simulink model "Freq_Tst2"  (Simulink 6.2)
settings: Solver=ode45  StartTime=0.0  StopTime=400  FixedStep=0.0005  MaxStep=0.002  RelTol=1e-3
undefined symbols (not defined in the file or in its folder): Aai, Aao, Af, Bai, Bao, Bf, Cai, Cao, Cf, Dai, Dao, Df, KJmix, KSmix

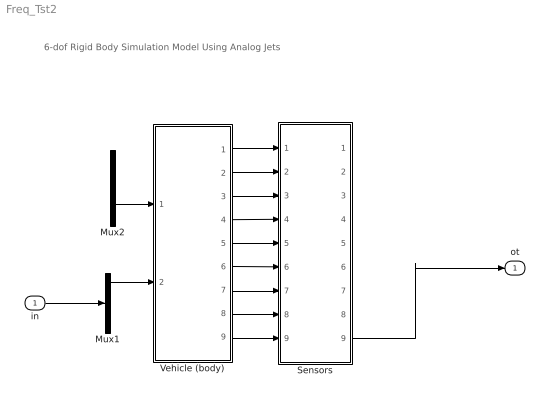
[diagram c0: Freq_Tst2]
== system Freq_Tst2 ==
  note: 6-dof Rigid Body Simulation Model Using Analog Jets
  in : Inport  Port=1  LatchInput=off
  Mux1 : Mux  Inputs=3
  Mux2 : Mux
  Sensors : Subsystem
  Vehicle (body) : Subsystem
  ot : Outport
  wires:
  Mux2/1 -> Vehicle (body)/1(Jet_PQR_Nz)
  Mux1/1 -> Vehicle (body)/2(Aer_pqr)
  in/1 -> Mux1/2
  Vehicle (body)/1(phi) -> Sensors/1(phi)
  Vehicle (body)/2(p) -> Sensors/2(pb)
  Vehicle (body)/3(r) -> Sensors/3(rb)
  Vehicle (body)/4(bet) -> Sensors/4(beta)
  Vehicle (body)/5(thet) -> Sensors/5(thet)
  Vehicle (body)/6(q) -> Sensors/6(q)
  Vehicle (body)/7(alf) -> Sensors/7(alfa)
  Vehicle (body)/8(Ny) -> Sensors/8(Ny)
  Vehicle (body)/9(Nz) -> Sensors/9(Nz)
  Sensors/9(Nzo) -> ot/1

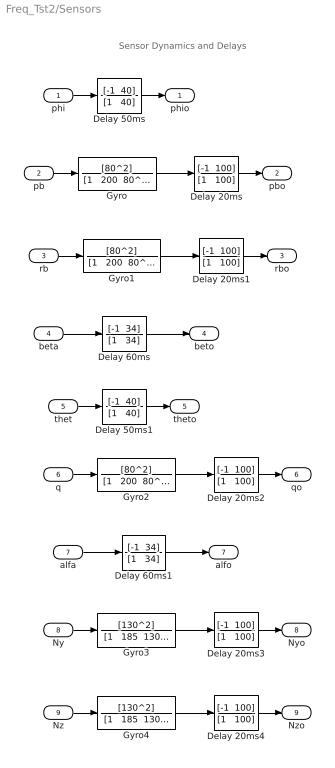
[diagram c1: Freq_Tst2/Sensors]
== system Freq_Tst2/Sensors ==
  note: Sensor Dynamics and Delays
  phi : Inport  Port=1  LatchInput=off
  pb : Inport  Port=2  LatchInput=off
  rb : Inport  Port=3  LatchInput=off
  beta : Inport  Port=4  LatchInput=off
  thet : Inport  Port=5  LatchInput=off
  q : Inport  Port=6  LatchInput=off
  alfa : Inport  Port=7  LatchInput=off
  Ny : Inport  Port=8  LatchInput=off
  Nz : Inport  Port=9  LatchInput=off
  Delay 20ms{,1..4} (5 alike) : TransferFcn  Numerator="[-1  100]"  Denominator="[1   100]"
  Delay 50ms : TransferFcn  Numerator="[-1  40]"  Denominator="[1   40]"
  Delay 50ms1 : TransferFcn  Numerator="[-1  40]"  Denominator="[1   40]"
  Delay 60ms : TransferFcn  Numerator="[-1  34]"  Denominator="[1   34]"
  Delay 60ms1 : TransferFcn  Numerator="[-1  34]"  Denominator="[1   34]"
  Gyro : TransferFcn  Numerator=[80^2]  Denominator="[1   200  80^2]"
  Gyro1 : TransferFcn  Numerator=[80^2]  Denominator="[1   200  80^2]"
  Gyro2 : TransferFcn  Numerator=[80^2]  Denominator="[1   200  80^2]"
  Gyro3 : TransferFcn  Numerator=[130^2]  Denominator="[1   185  130^2]"
  Gyro4 : TransferFcn  Numerator=[130^2]  Denominator="[1   185  130^2]"
  phio : Outport
  pbo : Outport  Port=2
  rbo : Outport  Port=3
  beto : Outport  Port=4
  theto : Outport  Port=5
  qo : Outport  Port=6
  alfo : Outport  Port=7
  Nyo : Outport  Port=8
  Nzo : Outport  Port=9
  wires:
  Gyro/1 -> Delay 20ms/1
  phi/1 -> Delay 50ms/1
  Delay 50ms/1 -> phio/1
  Delay 20ms/1 -> pbo/1
  pb/1 -> Gyro/1
  Gyro1/1 -> Delay 20ms1/1
  Delay 20ms1/1 -> rbo/1
  rb/1 -> Gyro1/1
  beta/1 -> Delay 60ms/1
  Delay 60ms/1 -> beto/1
  thet/1 -> Delay 50ms1/1
  Delay 50ms1/1 -> theto/1
  Gyro2/1 -> Delay 20ms2/1
  Delay 20ms2/1 -> qo/1
  q/1 -> Gyro2/1
  alfa/1 -> Delay 60ms1/1
  Delay 60ms1/1 -> alfo/1
  Gyro3/1 -> Delay 20ms3/1
  Delay 20ms3/1 -> Nyo/1
  Ny/1 -> Gyro3/1
  Gyro4/1 -> Delay 20ms4/1
  Delay 20ms4/1 -> Nzo/1
  Nz/1 -> Gyro4/1

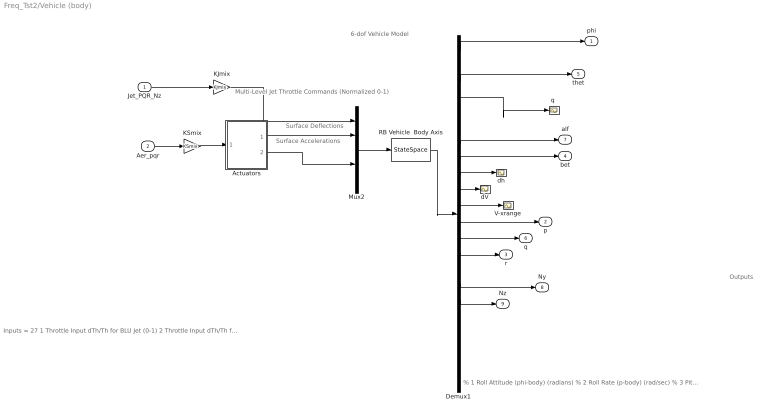
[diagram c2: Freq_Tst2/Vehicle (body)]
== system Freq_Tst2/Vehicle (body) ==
  note: Surface Deflections
  note: Multi-Level Jet Throttle Commands (Normalized 0-1)
  note: % 1 Roll Attitude (phi-body) (radians) % 2 Roll Rate (p-body) (rad/sec) % 3 Pitch Attitude (thet-bdy) (radians) % 4 Pitch Rate (q-body) (rad/sec) % 5 Yaw Attitude (psi-body) (radians) % 6 Yaw Rate (r-body) (rad/sec) % 7 Angle of attack, alfa, (radians) % 8 Angle of sideslip, beta, (radian) % 9 Change in Altitude, delta-h, (feet) % 10 Forward Acceleration (V-dot) (ft/sec) % 11 Cross Range Velocity (Vcr) (ft/sec) % 12 Rate-Gyro # 1, Roll Rate (Body) (rad/sec) % 13 Rate-Gyro # 2, Pitch Rate (Body) (rad/sec) % 14 Rate-Gyro # 3, Yaw Rate (Body) (rad/sec) % 15 Accelerom # 1, (along X), (ft/sec^2) Translat. Acceler % 16 Accelerom # 2, (along Y), (ft/sec^2) Translat. Acceler % 17 Accelerom # 3, (along Z), (ft/sec^2) Translat. Acceler % 18 Hinge Moment for Aero Surface # 1, (ft-lb) % 19 Hinge Moment for Aero Surface # 2, (ft-lb) % 20 Hinge Moment for Aero Surface # 3, (ft-lb) % 21 Hinge Moment for Aero Surface # 4, (ft-lb) % 22 Hinge Moment for Aero Surface # 5, (ft-lb)
  note: 6-dof Vehicle Model
  note: Outputs
  note: Surface Accelerations
  note: Inputs = 27 1 Throttle Input dTh/Th for BLU Jet (0-1) 2 Throttle Input dTh/Th for BRU Jet (0-1) 3 Throttle Input dTh/Th for BLD Jet (0-1) 4 Throttle Input dTh/Th for BRD Jet (0-1) 5 Throttle Input dTh/Th for BL+Y Jet (0-1) 6 Throttle Input dTh/Th for BR-Y Jet (0-1) 7 Throttle Input dTh/Th for FU Jet (0-1) 8 Throttle Input dTh/Th for FLD Jet (0-1) 9 Throttle Input dTh/Th for FRD Jet (0-1) 10 Throttle Input dTh/Th for FL+Y Jet (0-1) 11 Throttle Input dTh/Th for FR-Y Jet (0-1) 12 Left Outbrd Elevon Deflection (radians) 13 Left Inboard Elevon Deflection (radians) 14 Right Inbrd Elevon Deflection (radians) 15 Right Outbrd Elevon Deflection (radians) 16 Vertical Rudder Deflection (radians) 17 Left Outbrd Elevon Velocity (rad/sec) 18 Left Inboard Elevon Velocity (rad/sec) 19 Right Inbrd Elevon Velocity (rad/sec) 20 Right Outbrd Elevon Velocity (rad/sec) 21 Vertical Rudder Velocity (rad/sec) 22 Left Outbrd Elevon Acceleration (rad/s^2) 23 Left Inboard Elevon Acceleration (rad/s^2) 24 Right Inbrd Elevon Acceleration (rad/s^2) 25 Right Outbrd Elevon Acceleration (rad/s^2) 26 Vertical Rudder Acceleration (rad/s^2) 27 Gust Veloc. Azim,Elev=(45, 90) (deg)
  Jet_PQR_Nz : Inport  Port=1  LatchInput=off
  Aer_pqr : Inport  Port=2  LatchInput=off
  Actuators : Subsystem
  Demux1 : Demux  Outputs=22
  KJmix : Gain  Gain=KJmix  Multiplication=Matrix(K*u)
  KSmix : Gain  Gain=KSmix  Multiplication=Matrix(K*u)
  Mux2 : Mux  Inputs=[11, 5,5,5, 1]
  RB Vehicle  Body Axis : StateSpace  A=Af  B=Bf  C=Cf  D=Df
  V-xrange : Scope
  dV : Scope
  dh : Scope
  "q " : Scope
  phi : Outport
  p : Outport  Port=2
  r : Outport  Port=3
  bet : Outport  Port=4
  thet : Outport  Port=5
  q : Outport  Port=6
  alf : Outport  Port=7
  Ny : Outport  Port=8
  Nz : Outport  Port=9
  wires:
  Mux2/1 -> RB Vehicle  Body Axis/1
  Demux1/4 -> "q "/1
  Demux1/7 -> alf/1
  Demux1/8 -> bet/1
  Aer_pqr/1 -> KSmix/1
  Demux1/3 -> thet/1
  Demux1/1 -> phi/1
  Demux1/9 -> dh/1
  Demux1/10 -> dV/1
  Demux1/11 -> V-xrange/1
  Jet_PQR_Nz/1 -> KJmix/1
  KJmix/1 -> Mux2/1
  Demux1/12 -> p/1
  Demux1/13 -> q/1
  Demux1/14 -> r/1
  Demux1/17 -> Nz/1
  RB Vehicle  Body Axis/1 -> Demux1/1
  Actuators/1(delta) -> Mux2/2
  KSmix/1 -> Actuators/1(delcom)
  Demux1/16 -> Ny/1
  Actuators/2(delddot) -> Mux2/4

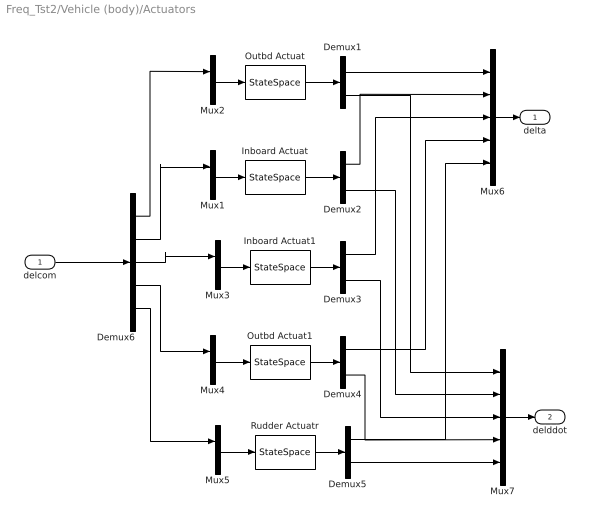
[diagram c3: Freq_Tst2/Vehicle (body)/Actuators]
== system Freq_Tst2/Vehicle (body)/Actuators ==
  delcom : Inport  Port=1  LatchInput=off
  Demux{1..5} (5 alike) : Demux  Outputs=3
  Demux6 : Demux  Outputs=5
  Inboard Actuat : StateSpace  A=Aai  B=Bai  C=Cai  D=Dai
  Inboard Actuat1 : StateSpace  A=Aai  B=Bai  C=Cai  D=Dai
  Mux{1..5} (5 alike) : Mux  Inputs=2
  Mux6 : Mux  Inputs=5
  Mux7 : Mux  Inputs=5
  Outbd Actuat : StateSpace  A=Aao  B=Bao  C=Cao  D=Dao
  Outbd Actuat1 : StateSpace  A=Aao  B=Bao  C=Cao  D=Dao
  Rudder Actuatr : StateSpace  A=Aai  B=Bai  C=Cai  D=Dai
  delta : Outport
  delddot : Outport  Port=2
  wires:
  Mux6/1 -> delta/1
  Mux7/1 -> delddot/1
  Mux1/1 -> Inboard Actuat/1
  Mux2/1 -> Outbd Actuat/1
  Mux3/1 -> Inboard Actuat1/1
  Mux4/1 -> Outbd Actuat1/1
  Mux5/1 -> Rudder Actuatr/1
  Outbd Actuat/1 -> Demux1/1
  Inboard Actuat/1 -> Demux2/1
  Inboard Actuat1/1 -> Demux3/1
  Outbd Actuat1/1 -> Demux4/1
  Rudder Actuatr/1 -> Demux5/1
  delcom/1 -> Demux6/1
  Demux6/1 -> Mux2/1
  Demux6/2 -> Mux1/1
  Demux6/3 -> Mux3/1
  Demux6/4 -> Mux4/1
  Demux6/5 -> Mux5/1
  Demux5/3 -> Mux7/5
  Demux4/3 -> Mux7/4
  Demux3/3 -> Mux7/3
  Demux2/3 -> Mux7/2
  Demux1/3 -> Mux7/1
  Demux1/1 -> Mux6/1
  Demux2/1 -> Mux6/2
  Demux3/1 -> Mux6/3
  Demux4/1 -> Mux6/4
  Demux5/1 -> Mux6/5
